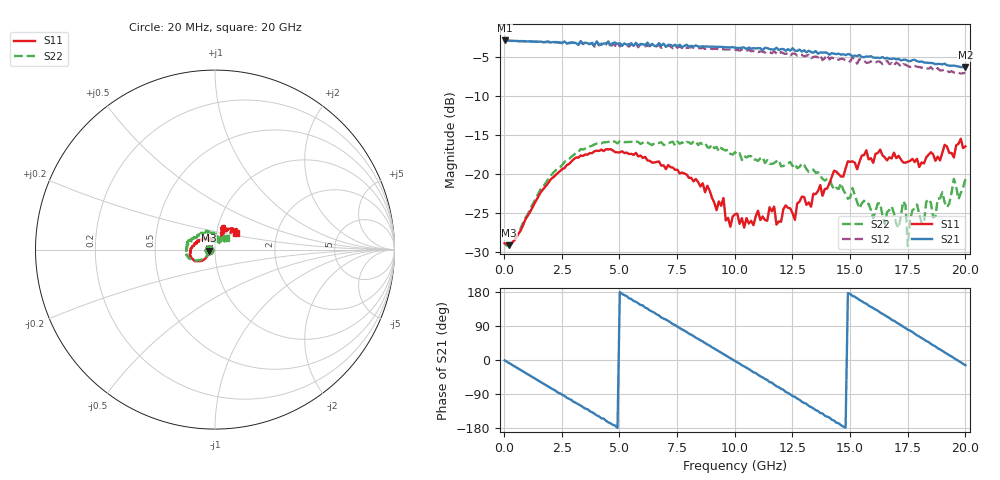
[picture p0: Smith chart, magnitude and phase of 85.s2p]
!Agilent Technologies,N5230A,US43500223,A.07.50.48
!Agilent N5230A: A.07.50.48
!Date: Wednesday, October 07, 2015 17:33:59
!Correction: S11(Full 2 Port(1,2))
!S21(Full 2 Port(1,2))
!S12(Full 2 Port(1,2))
!S22(Full 2 Port(1,2))
!S2P File: Measurements: S11, S21, S12, S22:
# Hz S  RI  R 50
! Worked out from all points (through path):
!   201 points, 20 MHz to 20 GHz, reference 50 ohm
!   highest |S21| = -2.94 dB at 20 MHz (marker M1); lowest = -6.4 dB at 20 GHz (marker M2)
!   group delay of S21, straight-line fit = 102 ps
!   lowest |S11| = -29.1 dB at 219.8 MHz (marker M3), VSWR 1.07, Z = 46.7 - j0.562 ohm
!   |S11| at or under -10 dB: start of sweep to end of sweep
!   |S22| runs from -29.3 to -15.8 dB; largest |S21 - S12| = 0.082
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2e7  -0.036 0.000297  0.7131 -0.00951  0.7121 -0.0114  -0.0359 0.000261
2.198e8  -0.0345 -0.00601  0.7035 -0.1025  0.7026 -0.1041  -0.0345 -0.0054
1.8182e9  -0.0622 -0.0563  0.2775 -0.641  0.2642 -0.6456  -0.0708 -0.0524
3.4166e9  -0.1151 -0.0607  -0.3867 -0.5624  -0.4069 -0.5388  -0.1318 -0.0558
4.9151e9  -0.1358 -0.0194  -0.677 -0.00574  -0.6974 0.0195  -0.1558 -0.0142
6.7133e9  -0.1152 0.0339  -0.3186 0.6072  -0.284 0.6045  -0.1559 0.0232
8.1119e9  -0.074 0.0581  0.2619 0.6053  0.2877 0.5775  -0.1507 0.0384
9.8102e9  -0.00946 0.0449  0.6412 0.053  0.6234 0.0128  -0.1208 0.0578
1.001e10  -0.00203 0.0551  0.6395 -0.0301  0.6186 -0.0646  -0.1232 0.061
1.17083e10  0.0265 0.0557  0.2642 -0.5636  0.2242 -0.5644  -0.0778 0.0877
1.18082e10  0.0254 0.0399  0.2267 -0.5992  0.1697 -0.5659  -0.0803 0.0896
1.34066e10  0.0317 0.0674  -0.3629 -0.4715  -0.3622 -0.4256  -0.0292 0.1023
1.49051e10  0.0525 0.1081  -0.5827 0.0358  -0.5274 0.0655  0.0114 0.0683
1.67033e10  0.0372 0.122  -0.1947 0.508  -0.1453 0.4818  0.00833 0.0581
1.71029e10  0.0493 0.1206  -0.0537 0.5409  -0.0113 0.5046  0.0023 0.0449
1.74026e10  0.0357 0.1122  0.0532 0.5352  0.0889 0.4915  0.0314 0.055
1.75025e10  0.0338 0.1147  0.0914 0.5207  0.126 0.4718  0.0192 0.0286
1.79021e10  0.0525 0.1132  0.2215 0.4763  0.2282 0.427  0.0185 0.0609
1.82018e10  0.0382 0.1101  0.3034 0.4167  0.3109 0.3671  0.00573 0.0479
1.84016e10  0.0606 0.1177  0.3487 0.3758  0.3428 0.3224  0.0243 0.0644
1.87013e10  0.0653 0.1021  0.4079 0.2932  0.3893 0.2428  0.0126 0.0519
2e10  0.1183 0.0918  0.4655 -0.1144  0.4185 -0.1435  0.0639 0.0669
